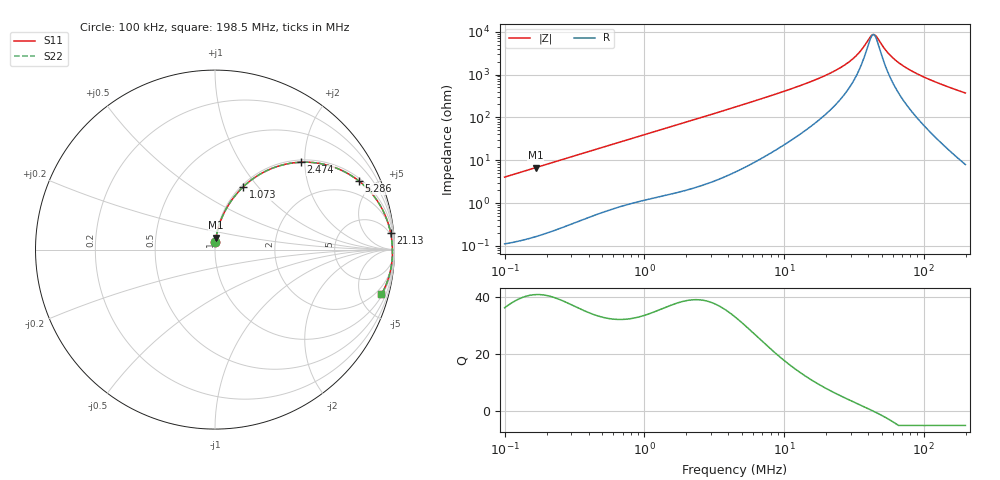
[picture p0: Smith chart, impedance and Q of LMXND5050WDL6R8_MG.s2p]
! LMXND5050WDL6R8_MG  S-PARAMETER MODEL  ( General Type )
! Model Generated by TAIYO YUDEN Corporation (http://www.ty-top.com)
! Version 1.0
! TAIYO YUDEN Control No. 191023NI43SB-FBB
! Copyright(c) 2019 TAIYO YUDEN CO.,LTD. All Rights Reserved.
! Product Description (link to TY-COMPAS)
! https://ds.yuden.co.jp/TYCOMPAS/or/detail?pn=LMXND5050WDL6R8MMG&u=M
! Products Name : Inductors
! Characteristics :
!  Inductance : 6.8 uH , SRF(min) : 28 MHz , DC Resistance(max) : 0.096 Ohm
!  Rated Current : Saturation :2200 mA , Temp Rise : 1600 mA
!  Case Size : 4.9 x 4.9 / 0.193 x 0.193 [mm/inch] , Thickness : 2.4 / 0.094 [mm/inch]
!  (Conditions: Temperature = 25 degC , DC Bias Current/Voltage = 0A / 0V)
! External Node Assignments :
!  1  o---GGG---o  2
! GND o---------o GND
! Frequency Range : 0.1MHz  -  198.534594MHz  [ 402 STEP ]
# MHz S RI R 50
! Freq[MHz].  S11 Real  S11 Imag  S21 Real  S21 Imag  S12 Real  S12 Imag  S22 Real  S22 Imag
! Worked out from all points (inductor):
!   401 points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, 100 kHz to 198.5 MHz, reference 50 ohm
!   read as one part in series: L = 6.43 uH near 103.9 kHz
!   highest Q = 40.8 at 167 kHz (marker M1), where L = 6.42 uH
!   self-resonance near 43.48 MHz
!   S11 on the Smith chart (normalised r, x): 100 kHz: 1.00, +0.08; 1.073 MHz: 1.02, +0.84; 2.474 MHz: 1.05, +1.92; 5.286 MHz: 1.14, +4.13; 21.13 MHz: 4, +21; 198.5 MHz: 1.16, -7.40
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0.1  0.00274 0.0403  0.9973 -0.0403  0.9973 -0.0403  0.00274 0.0403
0.166957  0.00614 0.0668  0.9939 -0.0668  0.9939 -0.0668  0.00614 0.0668
0.356769  0.0237 0.1388  0.9763 -0.1388  0.9763 -0.1388  0.0237 0.1388
0.667512  0.0715 0.2425  0.9285 -0.2425  0.9285 -0.2425  0.0715 0.2425
1.072936  0.1566 0.349  0.8434 -0.349  0.8434 -0.349  0.1566 0.349
1.272844  0.2039 0.389  0.7961 -0.389  0.7961 -0.389  0.2039 0.389
2.473636  0.4794 0.4869  0.5206 -0.4869  0.5206 -0.4869  0.4794 0.4869
4.541117  0.7513 0.4172  0.2487 -0.4172  0.2487 -0.4172  0.7513 0.4172
5.285906  0.8023 0.3819  0.1977 -0.3819  0.1977 -0.3819  0.8023 0.3819
8.65922  0.9124 0.2591  0.0876 -0.2591  0.0876 -0.2591  0.9124 0.2591
15.89665  0.968 0.1354  0.032 -0.1354  0.032 -0.1354  0.968 0.1354
21.13365  0.9788 0.091  0.0212 -0.091  0.0212 -0.091  0.9788 0.091
26.54053  0.9839 0.06  0.0161 -0.06  0.0161 -0.06  0.9839 0.06
31.48552  0.9863 0.0386  0.0137 -0.0386  0.0137 -0.0386  0.9863 0.0386
35.96028  0.9876 0.0226  0.0124 -0.0226  0.0124 -0.0226  0.9876 0.0226
41.07099  0.9883 0.00692  0.0117 -0.00692  0.0117 -0.00692  0.9883 0.00692
43.47794  0.9885 0.000235  0.0115 -0.000235  0.0115 -0.000235  0.9885 0.000235
46.02595  0.9886 -0.00647  0.0114 0.00647  0.0114 0.00647  0.9886 -0.00647
56.71438  0.9883 -0.0315  0.0117 0.0315  0.0117 0.0315  0.9883 -0.0315
68.57079  0.9868 -0.0556  0.0132 0.0556  0.0132 0.0556  0.9868 -0.0556
89.44651  0.9822 -0.0931  0.0178 0.0931  0.0178 0.0931  0.9822 -0.0931
198.5346  0.9274 -0.2491  0.0726 0.2491  0.0726 0.2491  0.9274 -0.2491
